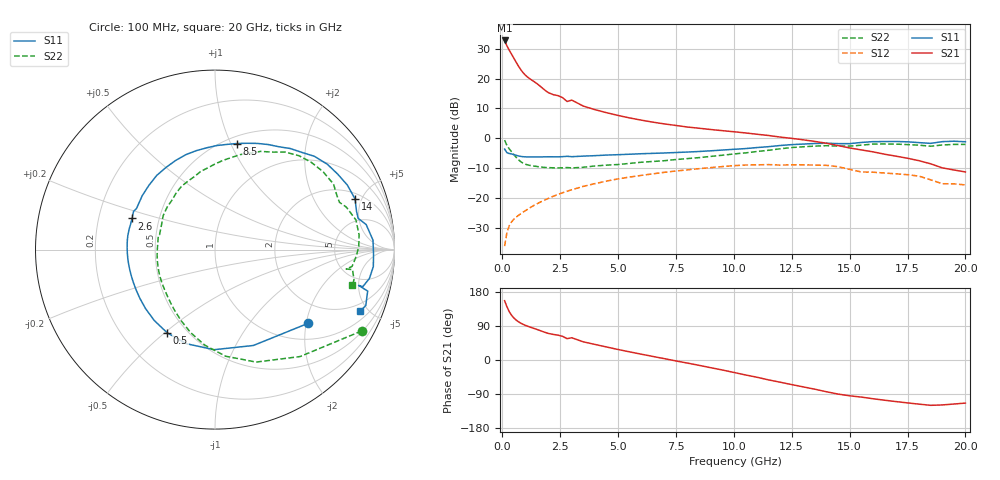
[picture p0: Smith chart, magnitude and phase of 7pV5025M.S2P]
! Infineon Technologies  Discrete & RF Semiconductors
! bfp620
! VCE = 0.50 V,  IC =  25 mA
! Common Emitter S-Parameters:  Sep 2002
# GHz  S  MA  R  50
!  f  S11  S21  S12  S22
! GHz  MAG  ANG  MAG  ANG  MAG  ANG  MAG  ANG
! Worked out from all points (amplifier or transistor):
!   59 points, 100 MHz to 20 GHz, reference 50 ohm
!   highest |S21| = 32.8 dB at 100 MHz (marker M1)
!   |S21| within 3 dB of that: start of sweep to 282.4 MHz
!   unconditionally stable (mu >= 1): 2.741 GHz to 2.874 GHz; 3.211 GHz to 10.09 GHz; 17.13 GHz to end of sweep
!   at 1 GHz: K = 0.77, MSG = 22.7 dB, |S12| = -24.2 dB
!   at 5.5 GHz: K = 1.05, MAG = 8.5 dB, |S12| = -13.0 dB
!   at 20 GHz: K = 1.64, MAG = -2.5 dB, |S12| = -15.6 dB
!   S11 on the Smith chart (normalised r, x): 100 MHz: 1.41, -2.06; 500 MHz: 0.39, -0.51; 2.6 GHz: 0.35, +0.16; 8.5 GHz: 0.57, +1.05; 14 GHz: 2.43, +4.41; 20 GHz: 1.49, -4.46
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0.1  0.6622 -38.3  43.51 156.6  0.0157 72.3  0.9347 -29.0
0.2  0.5754 -68.2  35.34 140.5  0.0266 59.8  0.7614 -51.5
0.3  0.5577 -90.5  29.91 127.7  0.0344 54.7  0.6673 -69.9
0.4  0.548 -106.9  25.61 118.1  0.04 51.8  0.5969 -84.3
0.5  0.5347 -119.8  21.92 110.9  0.0444 49.9  0.535 -96.2
0.6  0.5202 -130.5  18.76 105.3  0.0481 48.8  0.4812 -106.5
0.7  0.5079 -139.5  16.15 100.8  0.0515 48.3  0.438 -115.7
0.9  0.4935 -153.1  12.53 94.0  0.0583 48.1  0.3837 -130.7
1.1  0.4888 -162.1  10.54 89.0  0.0654 48.5  0.3593 -141.2
1.9  0.4914 173.1  6.152 71.8  0.0955 47.2  0.3252 -172.0
2.6  0.494 159.4  4.813 62.5  0.1229 43.2  0.3213 172.3
2.8  0.5013 154.8  4.14 56.3  0.1305 41.6  0.3252 166.0
3  0.4937 152.4  4.369 58.7  0.1383 40.1  0.3198 165.0
3.5  0.5047 143.4  3.468 47.9  0.1573 35.8  0.3287 155.0
5  0.5331 120.8  2.418 27.7  0.2097 21.8  0.365 131.1
7  0.5693 94.5  1.746 3.6  0.2703 2.2  0.4228 105.7
8.5  0.6034 78.4  1.477 -14.1  0.3112 -13.2  0.4765 90.1
10.5  0.6744 58.2  1.233 -39.4  0.3578 -36.9  0.5712 70.1
13.5  0.8204 26.0  0.888 -77.1  0.3571 -72.5  0.7424 35.8
14  0.8299 19.9  0.829 -83.8  0.3536 -79.5  0.7545 28.9
17  0.8872 -6.1  0.504 -109.7  0.255 -103.8  0.8012 1.2
20  0.8781 -22.9  0.274 -113.7  0.1662 -115.2  0.7913 -14.6
